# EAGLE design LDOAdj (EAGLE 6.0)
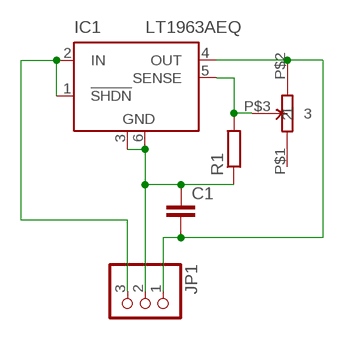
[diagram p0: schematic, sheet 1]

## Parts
C1  C2.5/4  [C2.5-4]
IC1  LT1963AEQ  [Q5-DD]
JP1  PINHD-1X3  [1X03]
R1  R-EU_0204/7  [0204/7]
U$1  TRIMPOTS  [TRIMPOTPACK]

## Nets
N$1: C1.1 IC1.3(GND) IC1.6(GND) JP1.2 R1.1
N$2: IC1.1(!SHDN) IC1.2(IN) JP1.3
N$3: C1.2 IC1.4(OUT) JP1.1 U$1.P$2
N$4: IC1.5(SENSE) R1.2 U$1.P$3
Unconnected: U$1.P$1

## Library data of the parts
C1 = capacitor-wima:C: CAPACITOR
IC1 = linear-technology:LT1963AEQ*: LT1963 1.5A, Low Noise, Fast Transient Response LDO Regulator Source: http://www.linear.com; MPN: LT1963AEQ; OC_FARNELL: 1273625; OC_NEWARK: 57M7427
JP1 = pinhead:PINHD-1X3: PIN HEADER
R1 = rcl:R-EU_: RESISTOR, European symbol
U$1 = larslib:TRIMPOTS: Grått trimpot 2.2kOhm PMR2K 9719 Mexico

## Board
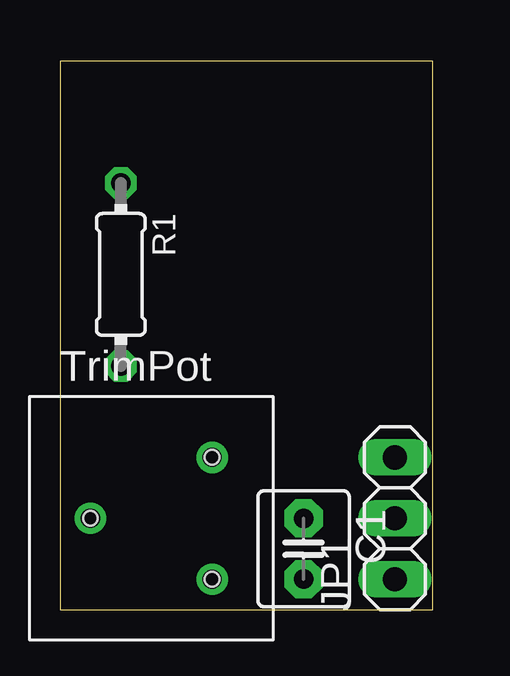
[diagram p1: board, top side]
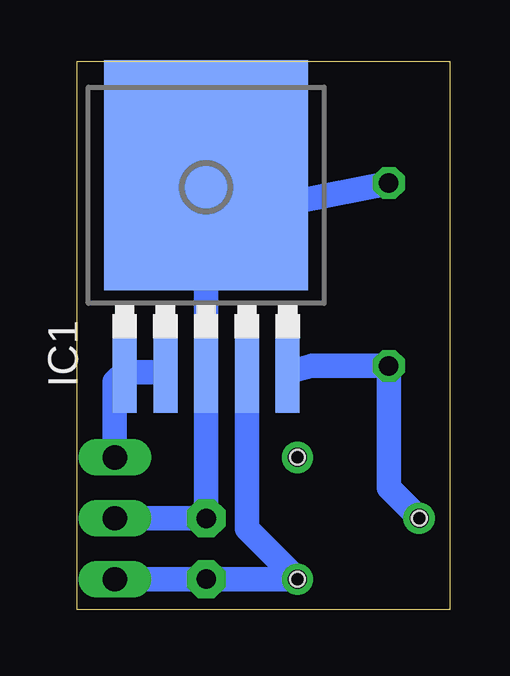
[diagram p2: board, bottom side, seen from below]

Size 15.54 x 22.85 mm. Coordinates in mm from the lower left corner, seen from the top.
Outline: 0,0 15.54,0 15.54,22.85 0,22.85 0,0
Copper layers (1*16): Top 0.035mm / dielectric 1.5mm / Bottom 0.035mm
Design rules: minimum track width 10mil, minimum drill 24mil, track to track 8mil, track to pad 8mil, pad to pad 8mil, via to via 8mil, smd to smd 8mil, copper to edge 40mil, drill to drill 8mil, minimum pad ring 10mil, minimum via ring 8mil, stop-mask expansion 4mil, vias tented up to drill 0mil, thermal gap 10mil

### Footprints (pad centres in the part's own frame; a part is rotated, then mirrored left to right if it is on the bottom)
C2.5-4 = drill 0.813 pad 1.6 octagon: 1 -1.27,0; 2 1.27,0
Q5-DD = smd 1 x 3.4: 1 -3.4,-7.875; 2 -1.7,-7.875; 3 0,-7.875; 4 1.7,-7.875; 5 3.4,-7.875 | smd 8.5 x 9.6: 6 0,0.325
1X03 = drill 1.016 long: 1 -2.54,0; 2 0,0; 3 2.54,0
0204/7 = drill 0.813 octagon: 1 -3.81,0; 2 3.81,0
TRIMPOTPACK = drill 0.8: P$1 2.54,5.08; P$2 2.54,0; P$3 -2.54,2.54 | hole 0.6: -2.54,2.54; 2.54,0; 2.54,5.08

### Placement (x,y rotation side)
C1  10.16,2.54 270 top
IC1  10.16,17.78 0 bottom
JP1  13.97,3.81 90 top
R1  2.54,13.97 270 top
U$1  3.81,1.27 0 top

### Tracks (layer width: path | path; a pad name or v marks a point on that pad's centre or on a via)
N$1
  Bottom 1.016: JP1.2 C1.1 IC1.3 10.16,16.51 9.53,17.14 | R1.1 8.89,16.51 9.53,17.14 | 9.53,17.14 10.16,17.78 IC1.6
N$2
  Bottom 1.016: JP1.3 13.97,9.49 IC1.1 IC1.2
N$3
  Bottom 1.016: JP1.1 C1.2 U$1.P$2 8.46,3.38 IC1.4
N$4
  Bottom 1.016: IC1.5 5.75,10.16 R1.2 2.54,5.08 U$1.P$3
